FUNCTION "AlarmsLoader" : VOID
TITLE =Alarms loader
VERSION : 0.1

BEGIN
NETWORK
TITLE =Fault control
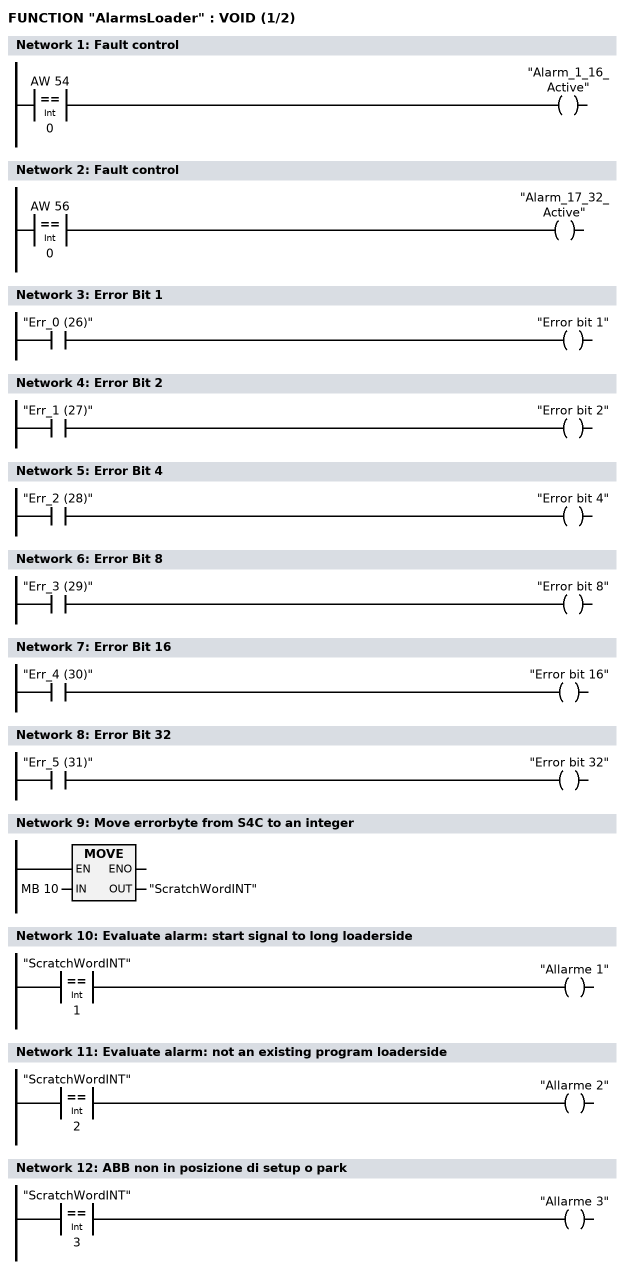
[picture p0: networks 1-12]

      L     AW    54;
      L     0;
      ==I   ;
      =     "Alarm_1_16_Active";
NETWORK
TITLE =Fault control

      L     AW    56;
      L     0;
      ==I   ;
      =     "Alarm_17_32_Active";
NETWORK
TITLE =Error Bit 1

      U     "Err_0 (26)";
      =     "Error bit 1";
NETWORK
TITLE =Error Bit 2

      U     "Err_1 (27)";
      =     "Error bit 2";
NETWORK
TITLE =Error Bit 4

      U     "Err_2 (28)";
      =     "Error bit 4";
NETWORK
TITLE =Error Bit 8

      U     "Err_3 (29)";
      =     "Error bit 8";
NETWORK
TITLE =Error Bit 16

      U     "Err_4 (30)";
      =     "Error bit 16";
NETWORK
TITLE =Error Bit 32

      U     "Err_5 (31)";
      =     "Error bit 32";
NETWORK
TITLE =Move errorbyte from S4C to an integer

      L     MB    10;
      T     "ScratchWordINT";
      NOP   0;
NETWORK
TITLE =Evaluate alarm: start signal to long loaderside

      L     "ScratchWordINT";
      L     1;
      ==I   ;
      =     "Allarme 1";
NETWORK
TITLE =Evaluate alarm: not an existing program loaderside

      L     "ScratchWordINT";
      L     2;
      ==I   ;
      =     "Allarme 2";
NETWORK
TITLE =ABB non in posizione di setup o park

      L     "ScratchWordINT";
      L     3;
      ==I   ;
      =     "Allarme 3";
NETWORK
TITLE =Programma non uguale tra ABB e Destacker
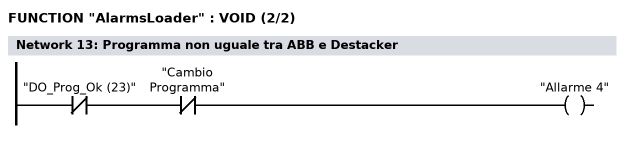
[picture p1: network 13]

      UN    "DO_Prog_Ok (23)";
      UN    "Cambio Programma";
      =     "Allarme 4";
NETWORK
TITLE =Anomalia inserzione motori ABB

      U(    ;
      UN    "Selezione manuale";
      U     "DO_Runch_Ok (5)";
      U     "DI_Mot_On (2)";
      UN    "DO_Mot_On_S (6)";
      L     S5T#2S;
      SE    "T19";
      NOP   0;
      NOP   0;
      NOP   0;
      U     "T19";
      )     ;
      S     "S4CLdNoMotorResponse";
      U     "Reset allarmi SH5";
      R     "S4CLdNoMotorResponse";
      U     "S4CLdNoMotorResponse";
      =     "Allarme 5";
NETWORK
TITLE =Programma ABB non in running
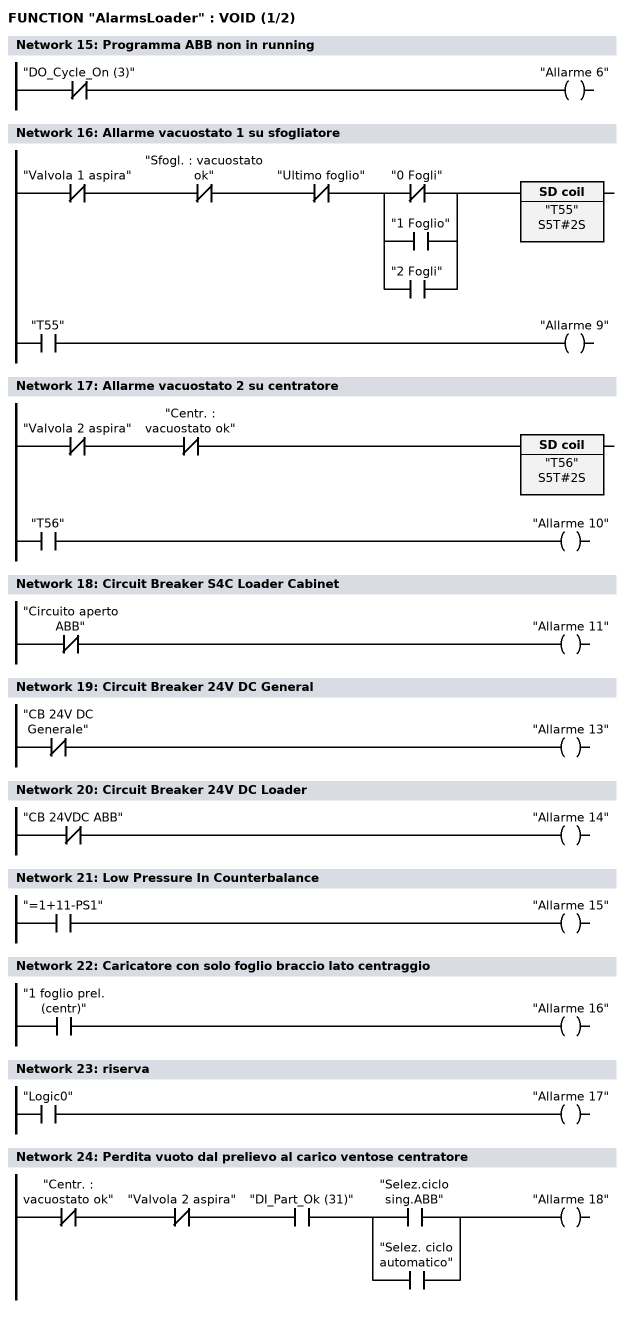
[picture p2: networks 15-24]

      UN    "DO_Cycle_On (3)";
      =     "Allarme 6";
NETWORK
TITLE =Allarme vacuostato 1 su sfogliatore

      UN    "Valvola 1 aspira";
      UN    "Sfogl. : vacuostato ok";
      UN    "Ultimo foglio";
      U(    ;
      ON    "0 Fogli";
      O     "1 Foglio";
      O     "2 Fogli";
      )     ;
      L     S5T#2S;
      SE    "T55";
      NOP   0;
      NOP   0;
      NOP   0;
      U     "T55";
      =     "Allarme 9";
NETWORK
TITLE =Allarme vacuostato 2 su centratore

      UN    "Valvola 2 aspira";
      UN    "Centr. : vacuostato ok";
      L     S5T#2S;
      SE    "T56";
      NOP   0;
      NOP   0;
      NOP   0;
      U     "T56";
      =     "Allarme 10";
NETWORK
TITLE =Circuit Breaker S4C Loader Cabinet

      UN    "Circuito aperto ABB";
      =     "Allarme 11";
NETWORK
TITLE =Circuit Breaker 24V DC General

      UN    "CB 24V DC Generale";
      =     "Allarme 13";
NETWORK
TITLE =Circuit Breaker 24V DC Loader

      UN    "CB 24VDC ABB";
      =     "Allarme 14";
NETWORK
TITLE =Low Pressure In Counterbalance

      U     "=1+11-PS1";
      =     "Allarme 15";
NETWORK
TITLE =Caricatore con solo foglio braccio lato centraggio

      U     "1 foglio prel. (centr)";
      =     "Allarme 16";
NETWORK
TITLE =riserva

      U     "Logic0";
      =     "Allarme 17";
NETWORK
TITLE =Perdita vuoto dal prelievo al carico ventose centratore

      UN    "Centr. : vacuostato ok";
      UN    "Valvola 2 aspira";
      U     "DI_Part_Ok (31)";
      U(    ;
      O     "Selez.ciclo sing.ABB";
      O     "Selez. ciclo automatico";
      )     ;
      =     "Allarme 18";
NETWORK
TITLE =Pressa non pronta per auto
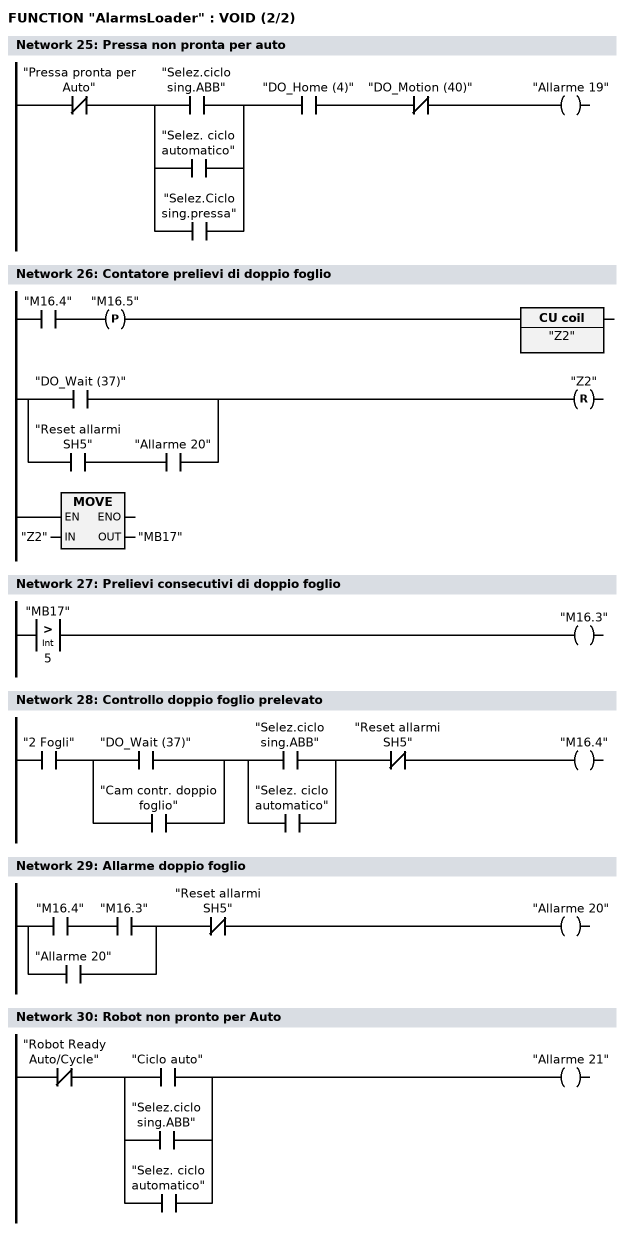
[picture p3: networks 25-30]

      UN    "Pressa pronta per Auto";
      U(    ;
      O     "Selez.ciclo sing.ABB";
      O     "Selez. ciclo automatico";
      O     "Selez.Ciclo sing.pressa";
      )     ;
      U     "DO_Home (4)";
      UN    "DO_Motion (40)";
      =     "Allarme 19";
NETWORK
TITLE = Contatore prelievi di doppio foglio

      U     "M16.4";
      FP    "M16.5";
      ZV    "Z2";
      BLD   101;
      NOP   0;
      NOP   0;
      U(    ;
      O     "DO_Wait (37)";
      O     ;
      U     "Reset allarmi SH5";
      U     "Allarme 20";
      )     ;
      R     "Z2";
      L     "Z2";
      T     "MB17";
      NOP   0;
      NOP   0;
NETWORK
TITLE =Prelievi consecutivi di doppio foglio

      L     "MB17";
      L     5;
      >I    ;
      =     "M16.3";
NETWORK
TITLE =Controllo doppio foglio prelevato

      U     "2 Fogli";
      U(    ;
      O     "DO_Wait (37)";
      O     "Cam contr. doppio foglio";
      )     ;
      U(    ;
      O     "Selez.ciclo sing.ABB";
      O     "Selez. ciclo automatico";
      )     ;
      UN    "Reset allarmi SH5";
      =     "M16.4";
NETWORK
TITLE =Allarme doppio foglio

      U(    ;
      U     "M16.4";
      U     "M16.3";
      O     "Allarme 20";
      )     ;
      UN    "Reset allarmi SH5";
      =     "Allarme 20";
NETWORK
TITLE =Robot non pronto per Auto

      UN    "Robot Ready Auto/Cycle";
      U(    ;
      O     "Ciclo auto";
      O     "Selez.ciclo sing.ABB";
      O     "Selez. ciclo automatico";
      )     ;
      =     "Allarme 21";
NETWORK
TITLE =No Part On Centering Station
//
//
      O(    ;
      UN    "P.E. su centratore";
      U     "DO_Home (4)";
      U(    ;
      O     "Condizioni ok per auto";
      O     "Ciclo auto";
      )     ;
      L     S5T#1S500MS;
      SE    "T75";
      NOP   0;
      NOP   0;
      NOP   0;
      U     "T75";
      )     ;
      O     ;
      U     "Allarme 22";
      UN    "Reset allarmi SH5";
      =     "Allarme 22";
NETWORK
TITLE =Loader Not In Production Position
//
//
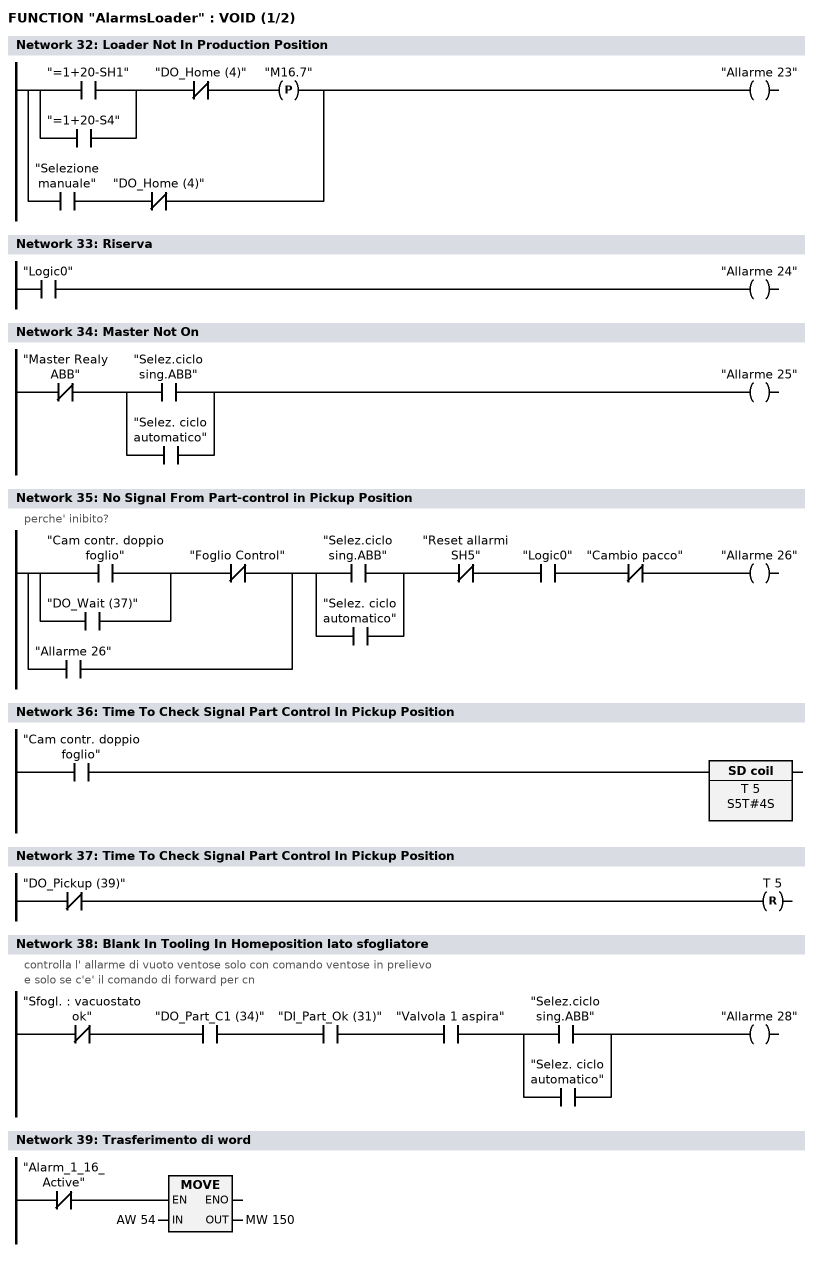
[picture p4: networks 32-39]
      U(    ;
      O     "=1+20-SH1";
      O     "=1+20-S4";
      )     ;
      UN    "DO_Home (4)";
      FP    "M16.7";
      O     ;
      U     "Selezione manuale";
      UN    "DO_Home (4)";
      =     "Allarme 23";
NETWORK
TITLE =Riserva

      U     "Logic0";
      =     "Allarme 24";
NETWORK
TITLE =Master Not On

      UN    "Master Realy ABB";
      U(    ;
      O     "Selez.ciclo sing.ABB";
      O     "Selez. ciclo automatico";
      )     ;
      =     "Allarme 25";
NETWORK
TITLE =No Signal From Part-control in Pickup Position
//perche' inibito?
      U(    ;
      U(    ;
      O     "Cam contr. doppio foglio";
      O     "DO_Wait (37)";
      )     ;
      UN    "Foglio Control";
      O     "Allarme 26";
      )     ;
      U(    ;
      O     "Selez.ciclo sing.ABB";
      O     "Selez. ciclo automatico";
      )     ;
      UN    "Reset allarmi SH5";
      U     "Logic0";
      UN    "Cambio pacco";
      =     "Allarme 26";
NETWORK
TITLE =Time To Check Signal Part Control In Pickup Position

      U     "Cam contr. doppio foglio";
      L     S5T#4S;
      SE    T      5;
NETWORK
TITLE =Time To Check Signal Part Control In Pickup Position

      UN    "DO_Pickup (39)";
      R     T      5;
NETWORK
TITLE =Blank In Tooling In Homeposition lato sfogliatore
//controlla l' allarme di vuoto ventose solo con comando ventose in prelievo
//e solo se c'e' il comando di forward per cn
//
      UN    "Sfogl. : vacuostato ok";
      U     "DO_Part_C1 (34)";
      U     "DI_Part_Ok (31)";
      U     "Valvola 1 aspira";
      U(    ;
      O     "Selez.ciclo sing.ABB";
      O     "Selez. ciclo automatico";
      )     ;
      =     "Allarme 28";
NETWORK
TITLE =Trasferimento di word

      UN    "Alarm_1_16_Active";
      SPBNB _001;
      L     AW    54;
      T     MW   150;
_001: NOP   0;
NETWORK
TITLE =Trasferimento di word
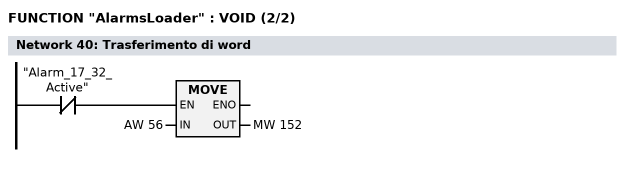
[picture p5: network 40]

      UN    "Alarm_17_32_Active";
      SPBNB _003;
      L     AW    56;
      T     MW   152;
_003: NOP   0;
END_FUNCTION

